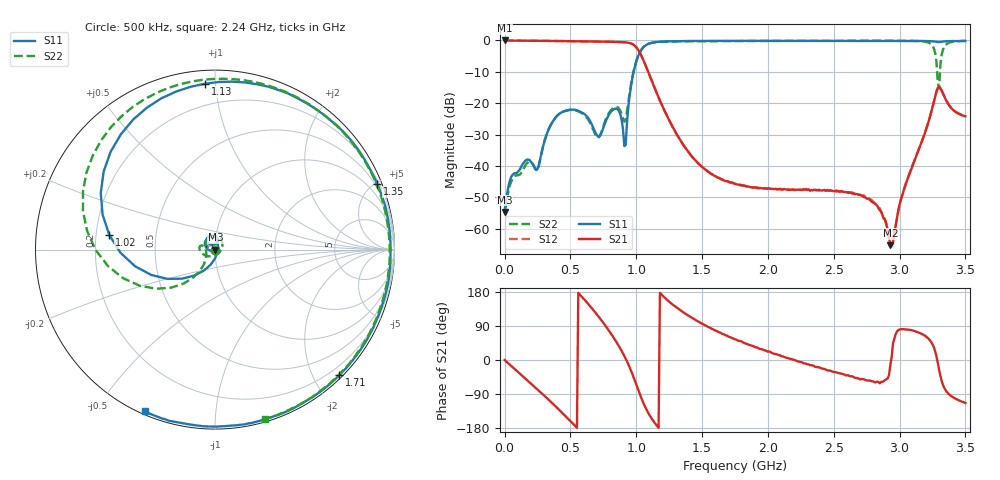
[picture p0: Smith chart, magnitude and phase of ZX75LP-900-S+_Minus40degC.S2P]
! Mini-Circuits
! S2P DATA File Format
! Type:LOW PASS FILTER
! Model: ZX75LP-900-S+
! All S Parameters are in dB deg format
! TEST CONDITIONS: INPUT POWER = 0 dBm @ Temperature = -40 deg C
! 401 Frequency points
# MHz S DB R 50
!FREQ	S11	S11_P	S21	S21_P	S12	S12_P	S22	S22_P
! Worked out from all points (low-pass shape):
!   401 points, 500 kHz to 3.5 GHz, reference 50 ohm
!   highest |S21| = -0.01 dB at 500 kHz (marker M1); lowest = -65.3 dB at 2.93 GHz (marker M2)
!   |S21| within 3 dB of the highest: start of sweep to 1.015 GHz
!   lowest |S11| = -54.7 dB at 500 kHz (marker M3), VSWR 1.00, Z = 50.2 + j0.0157 ohm
!   |S11| at or under -10 dB: start of sweep to 980.8 MHz
!   |S22| runs from -54.7 to -0.1 dB; largest |S21 - S12| = 0.0041
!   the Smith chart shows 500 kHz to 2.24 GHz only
!   S11 on the Smith chart (normalised r, x): 500 kHz: 1.00, +0.00; 1.02 GHz: 0.26, +0.06; 1.13 GHz: 0.07, +0.94; 1.35 GHz: 0.35, +5.11; 1.71 GHz: 0.05, -2.40; 2.24 GHz: 0.01, -0.66
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0.5  -54.72 4.9  -0.01 -0.1  -0.02 -0.2  -54.68 3.8
55  -43.17 -41.8  -0.04 -17.1  -0.05 -17.0  -44.65 -50.6
305  -31.88 -163.6  -0.14 -95.1  -0.14 -95.1  -31.79 -173.8
590  -23.06 84.1  -0.27 165.8  -0.27 165.8  -23.28 68.5
710  -30.64 96.1  -0.32 116.4  -0.32 116.4  -31.07 -50.8
790  -23.89 133.4  -0.40 78.9  -0.39 78.9  -23.32 -155.8
920  -33.31 -52.4  -0.61 3.5  -0.61 3.5  -25.24 -151.4
1020  -4.52 172.2  -3.36 -83.1  -3.33 -83.2  -4.38 -171.4
1130  -0.67 93.4  -14.18 -161.1  -14.18 -161.2  -0.67 114.9
1170  -0.44 75.8  -18.19 -178.8  -18.25 -178.9  -0.49 97.9
1350  -0.22 22.0  -32.79 127.7  -32.87 127.9  -0.30 47.8
1710  -0.13 -45.3  -45.36 60.7  -45.19 60.8  -0.22 -12.7
1760  -0.13 -52.4  -45.89 53.9  -45.75 55.4  -0.20 -19.5
2240  -0.15 -113.4  -47.56 -4.6  -47.52 -3.4  -0.14 -73.7
2340  -0.14 -124.7  -47.78 -14.4  -47.78 -13.5  -0.12 -83.9
2770  -0.17 -169.3  -50.51 -53.8  -50.72 -51.5  -0.07 -124.6
2920  -0.19 175.3  -62.89 -39.8  -62.70 -34.9  -0.07 -138.1
2930  -0.18 174.3  -65.27 -12.8  -64.82 -17.8  -0.08 -138.9
3210  -0.22 146.4  -27.33 59.5  -27.19 60.0  -0.55 -174.4
3290  -0.51 139.2  -15.23 -6.5  -15.21 -5.7  -13.21 150.4
3340  -0.32 136.0  -17.95 -73.8  -17.87 -72.4  -1.98 -134.8
3500  -0.20 121.3  -24.19 -113.2  -24.05 -112.2  -0.13 -169.3
